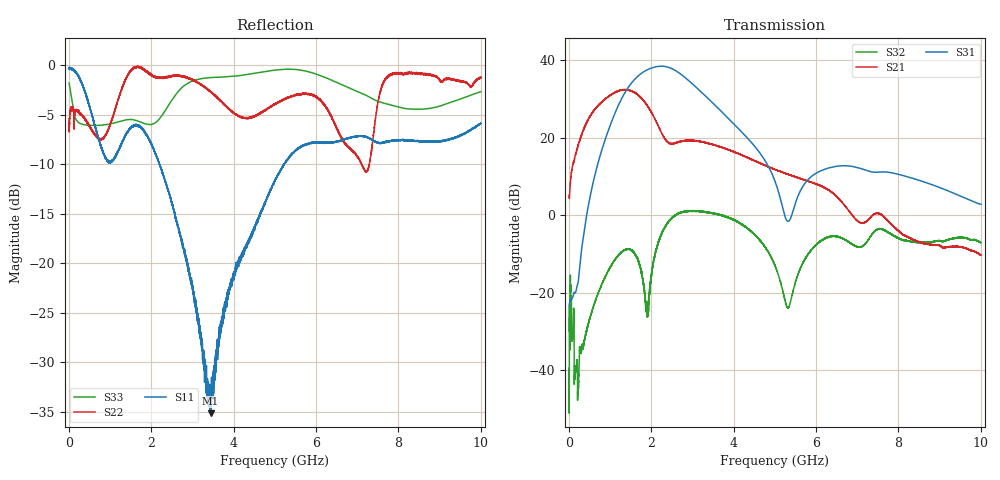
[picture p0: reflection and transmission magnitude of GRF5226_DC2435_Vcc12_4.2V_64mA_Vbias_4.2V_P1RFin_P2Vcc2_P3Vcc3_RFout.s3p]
!Keysight Technologies,N5245B,MY56052315,A.20.20.05
!Date: Friday, August 21, 2026 14:54:07
!Correction: S11(C  3-Port  )
!S12(C  3-Port  )
!S13(C  3-Port  )
!S21(C  3-Port  )
!S22(C  3-Port  )
!S23(C  3-Port  )
!S31(C  3-Port  )
!S32(C  3-Port  )
!S33(C  3-Port  )
!S3P File: Measurements: <S11,S12,S13>,
!<S21,S22,S23>,
!<S31,S32,S33>:
# Hz S  dB  R 50
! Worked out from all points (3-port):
!   9991 points, 10 MHz to 10 GHz, reference 50 ohm
!   strongest paths, dB at 10 MHz, 2.507 GHz, 5.005 GHz, 7.503 GHz, 10 GHz:
!     S31: -23.4, 37.8, 8.7, 11.1, 2.8
!     S21: 5.1, 18.4, 11.8, 0.5, -10.3
!     S32: -39.5, -0.7, -13.0, -3.6, -7.1
!   lowest |S11| = -35.2 dB at 3.443 GHz (marker M1), VSWR 1.04, Z = 49.5 + j1.66 ohm
!   |S11| at or under -10 dB: 2.202 GHz to 5.22 GHz (3.018 GHz wide, 81.3 % of centre); 5.221634 GHz to 5.231316 GHz (9.682 MHz wide, 0.185 % of centre); 5.233974 GHz to 5.234031 GHz (56.99 kHz wide, 0.00109 % of centre)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
1e7  -0.36 -1.7  -57.09 177.1  -50.20 150.2
     5.08 51.9  -5.41 -45.9  -55.28 146.8
     -23.43 -155.0  -39.53 59.0  -1.82 -56.3
6.06e8  -5.75 -92.3  -41.02 100.6  -66.99 173.0
        26.84 25.9  -6.80 169.6  -43.11 -61.9
        9.04 7.5  -23.32 0.8  -6.09 -169.1
1.14e9  -9.17 -104.6  -38.25 84.2  -61.06 110.2
        31.73 -35.8  -4.31 -161.7  -32.77 -137.6
        26.74 -60.3  -11.24 -65.8  -5.80 -171.1
1.525e9  -6.22 -137.8  -35.64 89.4  -56.40 85.1
         32.00 -90.7  -0.45 -176.4  -29.21 166.9
         34.10 -127.2  -8.97 -126.7  -5.49 -173.2
1.94e9  -7.37 167.7  -33.38 79.9  -58.38 79.1
        27.68 -147.4  -0.82 154.2  -30.89 118.2
        37.65 161.5  -21.94 -65.0  -6.00 -170.7
2.359e9  -12.02 120.6  -33.24 77.3  -56.66 57.4
         19.28 -160.9  -1.22 139.6  -31.70 114.8
         38.30 94.0  -2.66 -100.6  -4.48 -161.3
2.772e9  -18.36 80.7  -32.82 84.1  -57.71 82.4
         19.15 -149.7  -1.18 131.1  -29.11 92.2
         35.94 33.8  0.74 -157.5  -2.17 -168.9
3.443e9  -35.17 105.8  -29.90 89.5  -54.01 81.2
         18.28 -178.2  -2.74 131.7  -28.94 51.1
         29.46 -35.4  0.59 140.0  -1.26 172.1
5.005e9  -11.73 170.8  -26.59 70.3  -55.49 69.6
         11.78 122.8  -3.95 111.1  -36.37 -22.9
         8.73 -132.0  -12.96 35.2  -0.51 155.9
1e10  -5.87 107.2  -25.93 38.1  -55.47 28.5
      -10.29 52.9  -1.25 88.0  -30.24 -14.3
      2.80 130.9  -7.12 -33.4  -2.68 72.4
